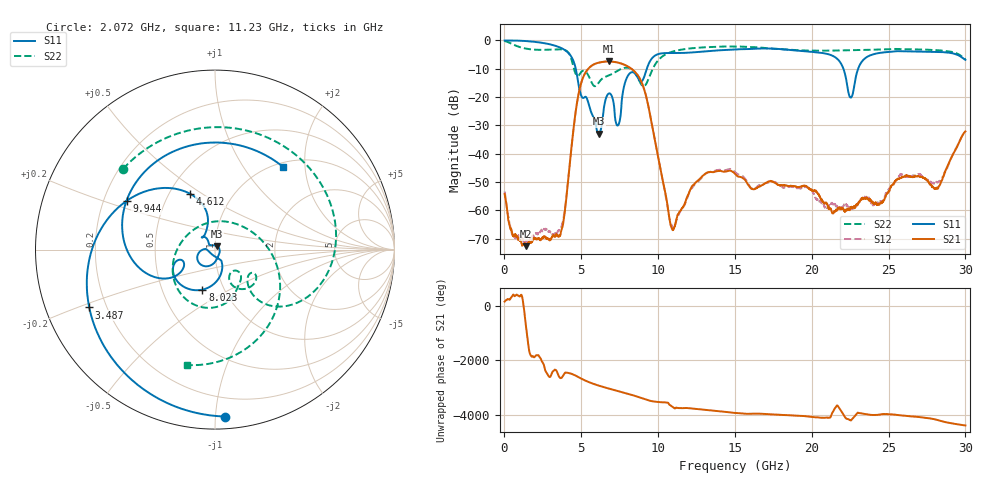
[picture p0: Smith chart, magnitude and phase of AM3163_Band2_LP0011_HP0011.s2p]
!Agilent Technologies,E8364B,MY43040894,A.07.50.67
!Agilent E8364B: A.07.50.67
!Date: Thursday, August 20, 2020 11:11:12
!Correction: S11(Full 2 Port(1,2))
!S21(Full 2 Port(1,2))
!S12(Full 2 Port(1,2))
!S22(Full 2 Port(1,2))
!S2P File: Measurements: S11, S21, S12, S22:
# Hz S  dB  R 50
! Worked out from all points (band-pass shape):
!   3201 points, 10 MHz to 30 GHz, reference 50 ohm
!   highest |S21| = -7.47 dB at 6.776 GHz (marker M1); lowest = -72.6 dB at 1.388 GHz (marker M2)
!   |S21| within 3 dB of the highest: 5.39 GHz to 8.361 GHz (2.971 GHz wide, 43.2 % of centre)
!   lowest |S11| = -32.9 dB at 6.13 GHz (marker M3), VSWR 1.05, Z = 51.2 + j1.97 ohm
!   |S11| at or under -10 dB: 4.639 GHz to 9.268 GHz (4.629 GHz wide, 66.6 % of centre); 22.06 GHz to 23.02 GHz (962.1 MHz wide, 4.27 % of centre)
!   |S22| runs from -16.2 to -0.2 dB; largest |S21 - S12| = 0.0035
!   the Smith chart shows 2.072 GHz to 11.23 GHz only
!   S11 on the Smith chart (normalised r, x): 2.072 GHz: 0.07, -1.06; 3.487 GHz: 0.14, -0.22; 4.612 GHz: 0.64, +0.45; 8.023 GHz: 0.79, -0.37; 9.944 GHz: 0.30, +0.24; 11.23 GHz: 1.08, +1.55
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1e7  -0.06 -2.9  -54.21 142.9  -53.34 169.6  -0.25 -11.1
5.910562e8  -0.08 -24.1  -69.18 40.2  -69.14 179.9  -1.55 -86.6
1.387666e9  -0.26 -57.2  -72.65 19.4  -70.76 133.2  -2.92 -168.4
2.071812e9  -0.61 -86.5  -70.28 -20.7  -68.18 157.7  -3.33 138.7
3.486966e9  -2.26 -155.3  -69.05 -20.2  -67.14 23.7  -3.16 39.9
4.611591e9  -9.38 113.9  -26.12 -44.7  -26.14 -45.0  -11.56 -46.3
5.014581e9  -19.72 122.2  -14.66 -164.8  -14.68 -165.1  -11.07 -34.6
6.129834e9  -32.94 58.6  -7.89 -56.1  -7.91 -56.3  -14.98 -43.2
6.776494e9  -18.82 -132.2  -7.47 -163.5  -7.47 -163.7  -12.44 -56.8
7.395038e9  -29.98 -121.8  -7.86 100.9  -7.91 100.7  -10.63 -74.4
8.022953e9  -12.61 -107.6  -9.20 3.7  -9.23 3.8  -9.69 -109.9
9.944188e9  -4.99 151.1  -39.52 64.8  -39.47 64.0  -7.46 -31.2
1.000979e10  -4.86 145.3  -41.33 61.3  -41.31 60.5  -7.03 -36.5
1.122813e10  -4.48 50.3  -62.43 -154.0  -63.13 -150.8  -3.59 -103.7
1.324309e10  -3.83 -68.3  -46.60 121.5  -46.63 125.0  -2.40 -173.6
1.5005e10  -3.20 -143.6  -47.14 20.4  -46.45 20.0  -2.18 128.1
1.769473e10  -3.00 94.1  -50.57 -45.9  -50.27 -46.1  -3.04 28.4
2.000958e10  -4.08 -29.7  -53.00 -128.4  -52.85 -129.1  -3.64 -51.8
2.253999e10  -20.22 -104.2  -58.95 103.5  -59.20 -57.1  -3.52 -122.5
2.500479e10  -4.12 -151.5  -53.28 -25.3  -52.83 -29.1  -3.20 177.5
2.818186e10  -4.09 109.7  -52.01 122.0  -50.22 120.9  -3.48 92.9
3e10  -6.88 42.3  -32.16 -78.7  -32.12 -78.5  -6.66 37.2
